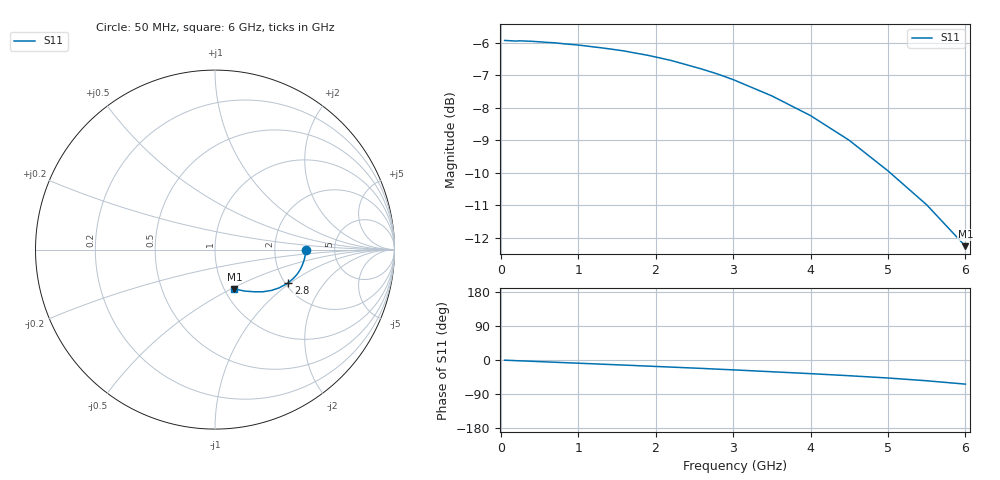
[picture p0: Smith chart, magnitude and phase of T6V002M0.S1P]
! SIEMENS Discrete & RF Semiconductors
! BAT62
! Si Schottky Diode in SOT143
! IF = 2 mA
! S-Parameters:  February  1997
# GHz  S  MA  R  50
!  f  S11
! GHz  MAG  ANG
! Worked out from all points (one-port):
!   34 points, 50 MHz to 6 GHz, reference 50 ohm
!   lowest |S11| = -12.3 dB at 6 GHz (marker M1), VSWR 1.65, Z = 55.8 - j25.9 ohm
!   |S11| at or under -10 dB: 5.029 GHz to end of sweep
!   S11 on the Smith chart (normalised r, x): 50 MHz: 3.04, -0.04; 2.8 GHz: 2.09, -0.96; 6 GHz: 1.12, -0.52
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0.05  0.5052 -0.5
0.15  0.5044 -1.3
0.2  0.5041 -1.8
0.25  0.5046 -2.2
0.3  0.5042 -2.5
0.4  0.5037 -3.4
0.7  0.501 -5.9
0.8  0.4995 -6.8
1  0.497 -8.4
1.1  0.4955 -9.3
1.3  0.4922 -11.0
1.4  0.4904 -11.8
1.5  0.4886 -12.7
1.6  0.4867 -13.5
1.7  0.4841 -14.3
1.8  0.4817 -15.3
2  0.4765 -17.0
2.2  0.4707 -18.7
2.4  0.4636 -20.5
2.6  0.4564 -22.2
2.8  0.4487 -24.2
3  0.4399 -26.0
3.5  0.4152 -31.0
4  0.3873 -36.0
4.5  0.3548 -41.5
5  0.3185 -47.5
5.5  0.2824 -54.8
6  0.2439 -63.7
